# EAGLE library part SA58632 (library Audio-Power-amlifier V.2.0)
The SA58632 is a two-channel audio amplifier in an HVQFN20 package. It provides power output of 2.2 W per channel with an 8 Ω load at 9 V supply. The internal circuit is comprised of two BTL (Bridge-Tied Load) amplifiers with a complementary PNP-NPN output stage and standby/mute logic. The SA58632 is housed in a 20-pin HVQFN package, which has an exposed die attach paddle enabling reduced thermal resistance and increased power dissipation
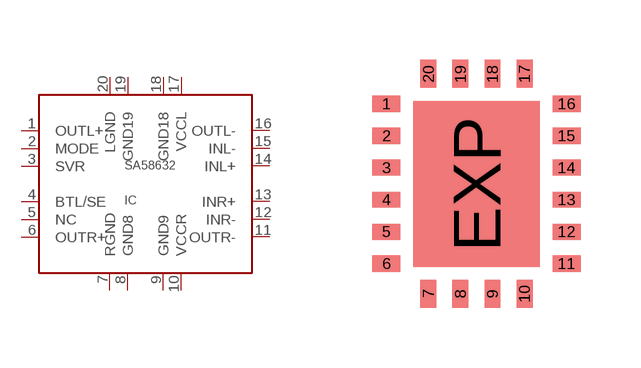
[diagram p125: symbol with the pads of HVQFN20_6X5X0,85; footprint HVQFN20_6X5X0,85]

Designator prefix IC

## SA58632SOT910-1  [HVQFN20_6X5X0,85]
1  OUTL+  out
2  MODE
3  SVR
4  BTL/SE
5  NC  nc
6  OUTR+  out
7  RGND  pwr
8  GND8  pwr
9  GND9  pwr
10  VCCR  pwr
11  OUTR-  out
12  INR-  in
13  INR+  in
14  INL+  in
15  INL-  in
16  OUTL-  out
17  VCCL  pwr
18  GND18  pwr
19  GND19  pwr
20  LGND  pwr

## Footprint HVQFN20_6X5X0,85 (pad centres in mm)
HVQFN20: plastic thermal enhanced very thin quad flat package; no leads; 20 terminals; body 6 x 5 x 0.85 mm SOT910-1
smd 0.7 x 0.4: 1 -2.25,2; 2 -2.25,1.2; 3 -2.25,0.4; 4 -2.25,-0.4; 5 -2.25,-1.2; 6 -2.25,-2; 11 2.25,-2; 12 2.25,-1.2; 13 2.25,-0.4; 14 2.25,0.4; 15 2.25,1.2; 16 2.25,2
smd 0.4 x 0.7: 7 -1.2,-2.75; 8 -0.4,-2.75; 9 0.4,-2.75; 10 1.2,-2.75; 17 1.2,2.75; 18 0.4,2.75; 19 -0.4,2.75; 20 -1.2,2.75
smd 3.15 x 4.15: EXP 0,-0.01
